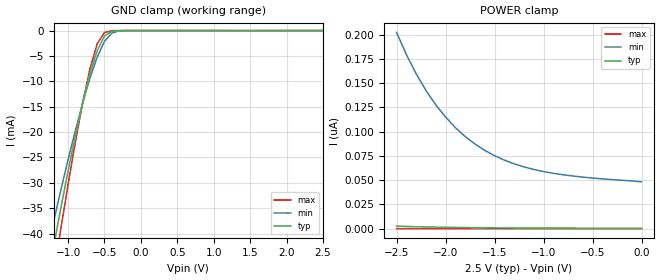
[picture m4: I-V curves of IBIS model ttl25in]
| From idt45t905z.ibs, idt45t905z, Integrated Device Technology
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|   Model ttl25in
[Model]   ttl25in
Model_type   Input
Polarity   Non-Inverting
Vinl =  0.70000V
Vinh =  1.70000V
Vmeas =  1.25000V
C_comp   5.00000pF   5.00000pF   5.00000pF
[Temperature Range]   45.00000   0.14000k   -30.00000
[Voltage Range]   2.50000V   2.30000V   2.70000V
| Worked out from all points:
|   GND clamp passes 1 mA (typ) near -0.49 V on its own axis
[GND_clamp]
| voltage   I(typ)   I(min)   I(max)
-2.5V     -150.1mA   -128.5mA   -173mA
-1.3V     -50.47mA   -44.23mA   -57.51mA
-1.2V     -42.64mA   -37.76mA   -48.2mA
-1.1V     -35.02mA   -31.48mA   -39.1mA
-900mV    -20.73mA   -19.68mA   -21.96mA
-800mV    -14.28mA   -14.3mA    -14.26mA
-700mV    -8.553mA   -9.407mA   -7.567mA
-600mV    -3.939mA   -5.223mA   -2.609mA
-500mV    -1.074mA   -2.122mA   -375.8uA
-400mV    -131.3uA   -507.1uA   -20.31uA
-300mV    -7.825uA   -67.79uA   -384.6nA
2.5V      443.6pA    49.9nA     1.135pA
[POWER_clamp]
| voltage   I(typ)   I(min)   I(max)
-2.5V     2.616nA    202.4nA    8.153pA
-2.4V     2.294nA    179.5nA    7.17pA
-2.3V     2.014nA    159.7nA    6.305pA
-2.2V     1.772nA    142.5nA    5.573pA
-2.1V     1.564nA    127.7nA    4.925pA
-1.9V     1.231nA    104.2nA    3.911pA
-1.8V     1.1nA      95.05nA    3.496pA
-1.6V     895.6pA    80.73nA    2.854pA
-1.3V     696.3pA    66.86nA    2.22pA
-1V       581.4pA    58.89nA    1.825pA
-600mV    500.6pA    53.16nA    1.519pA
0V        443.6pA    48.28nA    1.265pA
